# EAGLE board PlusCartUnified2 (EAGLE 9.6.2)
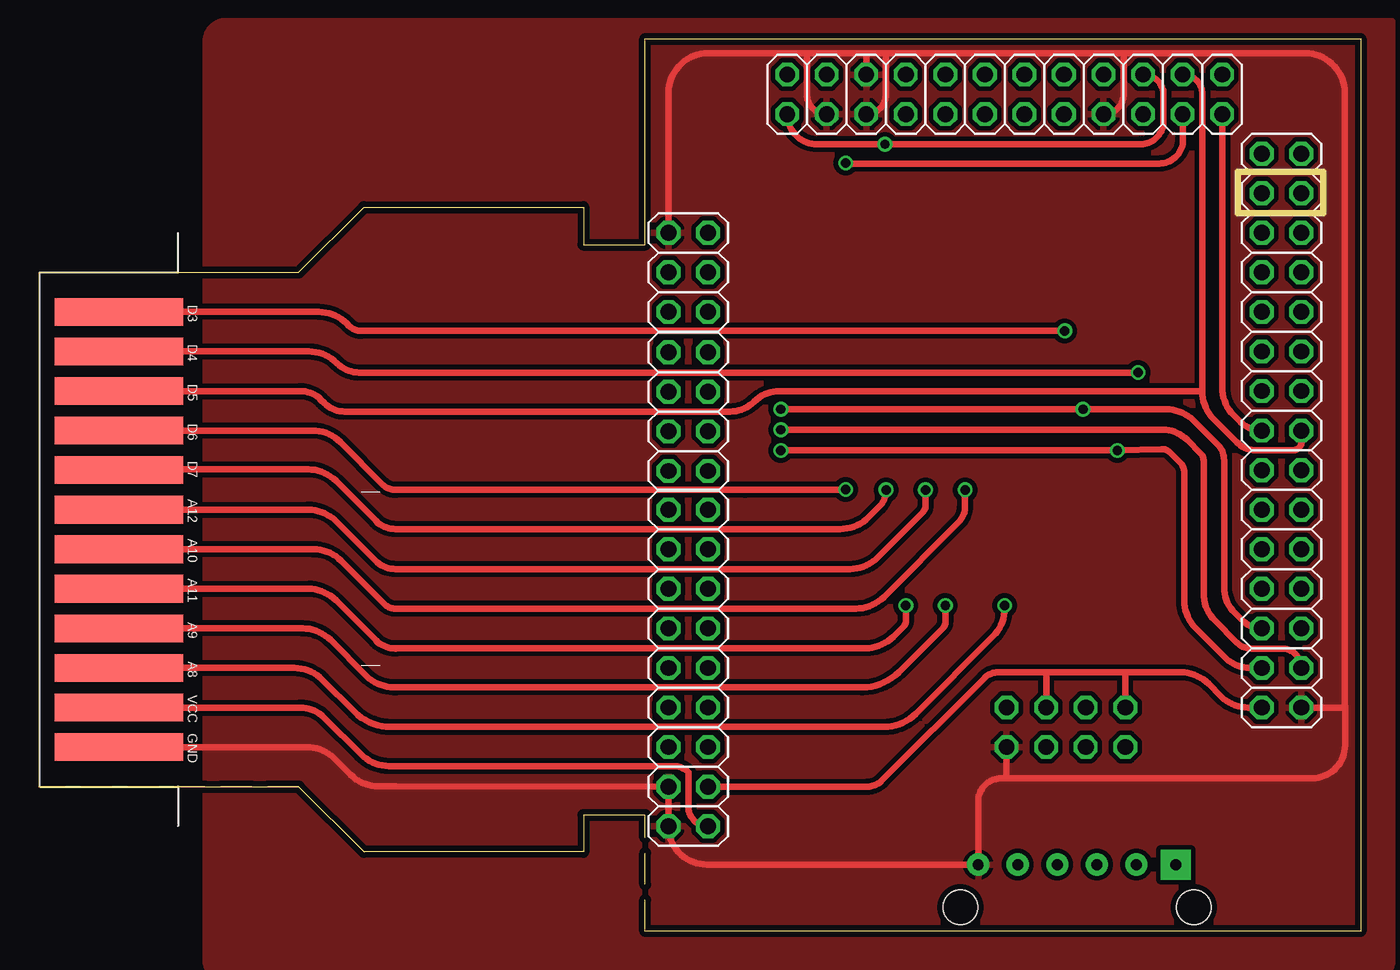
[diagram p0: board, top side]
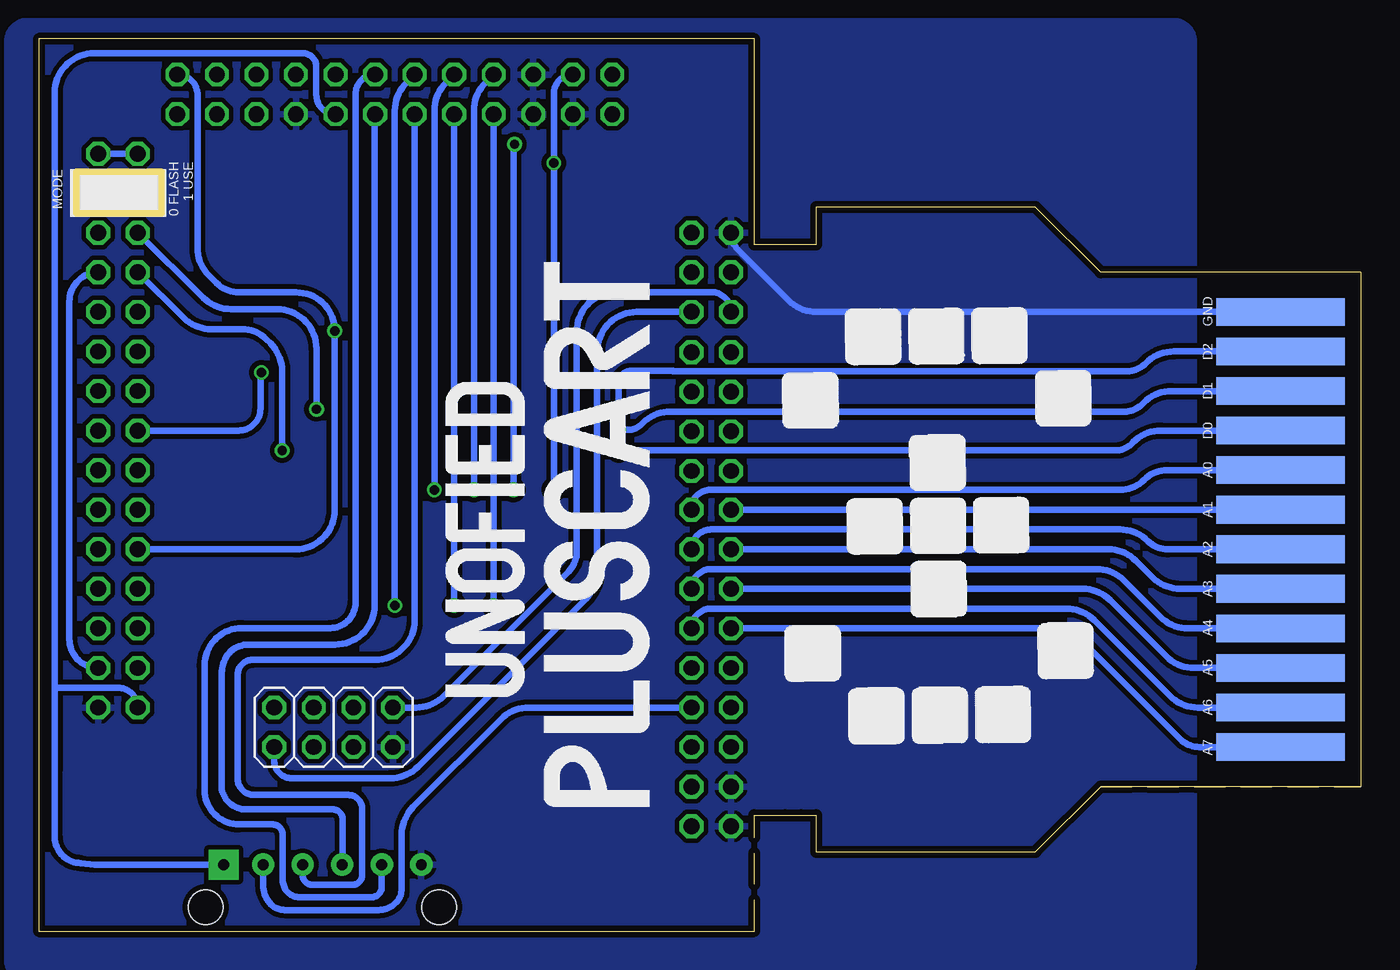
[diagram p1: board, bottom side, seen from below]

Size 84.89 x 57.28 mm. Coordinates in mm from the lower left corner, seen from the top.
Outline: 38.94,7.44 34.98,7.44
Outline: 34.98,7.44 34.98,5.08 20.88,5.08 16.69,9.27
Outline: 0,9.27 0,42.29 16.69,42.29 20.88,46.48 34.98,46.48 34.98,44.07 38.94,44.07 38.94,57.28 84.89,57.28 84.89,0 38.94,0 38.94,7.44
Outline: 0,9.27 16.69,9.27
Outline: 38.94,7.44 34.98,7.44
Outline: 16.69,9.27 0,9.27
Copper layers (1*16): Top 0.0356mm / dielectric 1.5011mm / Bottom 0.0356mm
Design rules "OSHPark2layer": minimum track width 6mil, minimum drill 13mil, track to track 6mil, track to pad 6mil, pad to pad 6mil, via to via 6mil, smd to smd 6mil, copper to edge 15mil, drill to drill 6mil, minimum pad ring 7mil, minimum via ring 7mil, stop-mask expansion 3mil, vias tented up to drill 0mil, thermal gap 10mil
Milling: 4 lines

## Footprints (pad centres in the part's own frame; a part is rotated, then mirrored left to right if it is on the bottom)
24PINEDGE-254MM = smd 1.778 x 8.255: 1-A -22.86,-7.62; 2-A -20.32,-7.62; 3-A -17.78,-7.62; 4-A -15.24,-7.62; 5-A -12.7,-7.62; 6-A -10.16,-7.62; 7-A -7.62,-7.62; 8-A -5.08,-7.62; 9-A -2.54,-7.62; 10-A 0,-7.62; 11-A 2.54,-7.62; 12-A 5.08,-7.62 | smd 1.778 x 8.255 bottom: 1-B -22.86,-7.62; 2-B -20.32,-7.62; 3-B -17.78,-7.62; 4-B -15.24,-7.62; 5-B -12.7,-7.62; 6-B -10.16,-7.62; 7-B -7.62,-7.62; 8-B -5.08,-7.62; 9-B -2.54,-7.62; 10-B 0,-7.62; 11-B 2.54,-7.62; 12-B 5.08,-7.62
2X02 = drill 1.016 octagon: 1 -1.27,-1.27; 2 -1.27,1.27; 3 1.27,-1.27; 4 1.27,1.27
2X04 = drill 1.016 octagon: 1 -3.81,-1.27; 2 -3.81,1.27; 3 -1.27,-1.27; 4 -1.27,1.27; 5 1.27,-1.27; 6 1.27,1.27; 7 3.81,-1.27; 8 3.81,1.27
2X03 = drill 1.016 octagon: 1 -2.54,-1.27; 2 -2.54,1.27; 3 0,-1.27; 4 0,1.27; 5 2.54,-1.27; 6 2.54,1.27
2X09 = drill 1.016 octagon: 1 -10.16,-1.27; 2 -10.16,1.27; 3 -7.62,-1.27; 4 -7.62,1.27; 5 -5.08,-1.27; 6 -5.08,1.27; 7 -2.54,-1.27; 8 -2.54,1.27; 9 0,-1.27; 10 0,1.27; 11 2.54,-1.27; 12 2.54,1.27; 13 5.08,-1.27; 14 5.08,1.27; 15 7.62,-1.27; 16 7.62,1.27; 17 10.16,-1.27; 18 10.16,1.27
2X08 = drill 1.016 octagon: 1 -8.89,-1.27; 2 -8.89,1.27; 3 -6.35,-1.27; 4 -6.35,1.27; 5 -3.81,-1.27; 6 -3.81,1.27; 7 -1.27,-1.27; 8 -1.27,1.27; 9 1.27,-1.27; 10 1.27,1.27; 11 3.81,-1.27; 12 3.81,1.27; 13 6.35,-1.27; 14 6.35,1.27; 15 8.89,-1.27; 16 8.89,1.27
2X07 = drill 1.016 octagon: 1 -7.62,-1.27; 2 -7.62,1.27; 3 -5.08,-1.27; 4 -5.08,1.27; 5 -2.54,-1.27; 6 -2.54,1.27; 7 0,-1.27; 8 0,1.27; 9 2.54,-1.27; 10 2.54,1.27; 11 5.08,-1.27; 12 5.08,1.27; 13 7.62,-1.27; 14 7.62,1.27
MICROSD_FOOTPRINT = drill 0.7 pad 1.93 square: 3V3 -15.24,6.35 | drill 0.7 pad 1.422: CLK -15.24,-1.27; CS -15.24,3.81; GND -15.24,-6.35; MISO -15.24,-3.81; MOSI -15.24,1.27 | hole 2.2: -12.5,7.5; -12.5,-7.5

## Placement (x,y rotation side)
CON3  A2600  [24PINEDGE-254MM]  12.75,34.67 90 bottom
JP1  0  [2X02]  41.71,8 270 top
JP2  0  [2X04]  41.71,23.24 270 top
JP3  0  [2X03]  41.71,42.29 270 top
JP4  0  [2X09]  58.22,53.72 180 top
JP5  0  [2X08]  79.81,23.24 90 top
JP6  0  [2X04]  65.96,13.08 0 bottom
JP7  0  [2X03]  41.71,14.35 270 top
JP8  0  [2X04]  41.71,33.35 270 top
JP10  0  [2X03]  73.46,53.72 0 top
JP11  0  [2X07]  79.81,42.29 270 top
SD1  MICROSDMICROSD2  [MICROSD_FOOTPRINT]  66.68,-10.97 270 top

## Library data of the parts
CON3 = con-edge
JP1-JP6 = pinhead
JP7 JP8 JP10 JP11 = pinhead@1
SD1 = MICROSD

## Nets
+3V3: JP1.2 JP4.4 JP5.2 JP6.2 JP6.6 SD1.3V3
A0: CON3.8-A JP2.2
A1: CON3.7-A JP2.1
A2: CON3.6-A JP2.4
A3: CON3.5-A JP2.3
A4: CON3.4-A JP2.6
A5: CON3.3-A JP2.5
A6: CON3.2-A JP2.8
A7: CON3.1-A JP2.7
A8: CON3.3-B JP4.7
A9: CON3.4-B JP4.10
A10: CON3.6-B JP4.9
A11: CON3.5-B JP4.12
A12: CON3.7-B JP4.11
CLK: JP4.6 SD1.CLK
CS: JP7.4 SD1.CS
D0: CON3.9-A JP5.4 JP11.7
D1: CON3.10-A JP5.3 JP11.8
D2: CON3.11-A JP5.6 JP11.5
D3: CON3.12-B JP5.10 JP10.6
D4: CON3.11-B JP5.16 JP10.5
D5: CON3.10-B JP5.15 JP10.4
D6: CON3.9-B JP4.15 JP10.3
D7: CON3.8-B JP4.18 JP10.2
GND: CON3.1-B CON3.12-A JP1.1 JP1.3 JP3.1 JP4.2 JP4.13 JP4.14 JP4.16 JP5.1 JP6.7 SD1.GND
MISO: JP4.5 SD1.MISO
MOSI: JP4.8 SD1.MOSI
SHORT: JP11.1 JP11.2
USART1_RX: JP3.5 JP6.8
USART1_TX: JP3.6 JP6.1
VCC: CON3.2-B JP1.4

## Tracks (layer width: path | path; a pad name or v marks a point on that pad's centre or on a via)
+3V3
  Top 0.406: JP1.2 53.22,9.27 arc45 54.12,9.64 60.71,16.24 arc-45 61.61,16.61 64.78,16.61 | JP5.2 77.67,14.35 arc-45 75.92,15.07 75.13,15.87 arc45 73.33,16.61 69.84,16.61 | 64.78,16.61 69.84,16.61 | JP6.6 64.69,16.39 arc-45 64.78,16.61 | JP6.2 69.77,16.44 arc-45 69.84,16.61
  Bottom 0.406: JP4.4 arc90 67.07,53.68 67.07,55.5 arc-90 67.94,56.37 81.33,56.37 arc-90 83.87,53.83 83.87,15.62 | 83.87,15.62 83.87,10.37 arc90 83.86,10.36 83.86,6.02 arc-90 82.21,4.37 81.3,4.27 SD1.3V3 | JP5.2 arc-90 79.81,15.62 83.87,15.62
A0
  Bottom 0.406: JP2.2 42.98,27.12 arc90 41.77,28.33 15.47,28.33 arc-45 13.89,28.98 arc45 12.42,29.59 CON3.8-A
A1
  Bottom 0.406: JP2.1 CON3.7-A
A2
  Bottom 0.406: JP2.4 arc90 41.71,25.78 15.45,25.78 arc45 13.66,25.04 arc-45 12.39,24.51 CON3.6-A
A3
  Bottom 0.406: JP2.3 16.22,24.51 arc45 14.42,23.77 13.37,22.71 arc-45 11.57,21.97 CON3.5-A
A4
  Bottom 0.406: JP2.6 arc90 41.71,23.24 16.98,23.24 arc45 15.18,22.5 12.86,20.18 arc-45 11.06,19.43 CON3.4-A
A5
  Bottom 0.406: JP2.5 17.87,21.97 arc45 16.07,21.23 12.48,17.64 arc-45 10.68,16.89 CON3.3-A
A6
  Bottom 0.406: JP2.8 arc90 41.71,20.7 18.91,20.7 arc45 17.11,19.96 12.25,15.1 arc-45 10.45,14.35 CON3.2-A
A7
  Bottom 0.406: JP2.7 19.75,19.43 arc45 17.95,18.69 11.58,12.32 arc-45 10.36,11.81 CON3.1-A
A8  (via drill 0.6)
  Top 0.406: CON3.3-B 16.4,16.89 arc-45 18.19,16.15 20.26,14.08 arc45 22.6,13.11 54.28,13.11 arc45 56.32,13.95 61.28,18.92 arc45 62.03,20.71 v62.03,20.9
  Bottom 0.406: JP4.7 61.28,54.47 arc-45 62.03,52.67 v62.03,20.9
A9  (via drill 0.6)
  Top 0.406: v58.22,20.9 58.22,19.84 arc-45 58.05,19.45 55.23,16.62 arc-45 52.89,15.65 22.91,15.65 22.82,15.65 arc-45 21.02,16.39 18.73,18.69 arc45 16.93,19.43 CON3.4-B
  Bottom 0.406: JP4.10 v58.22,20.9
A10  (via drill 0.6)
  Top 0.406: v59.49,28.32 59.49,27.28 arc-45 59.06,26.24 54.26,21.45 arc-45 52.47,20.7 22.91,20.7 arc-45 22.17,21.01 19.41,23.77 arc45 17.62,24.51 CON3.6-B
  Bottom 0.406: JP4.9 58.74,54.47 arc-45 59.49,52.67 v59.49,28.32
A11  (via drill 0.6)
  Top 0.406: v55.68,20.9 55.68,19.89 arc-45 55.55,19.59 54.87,18.91 arc-45 53.07,18.16 22.97,18.16 arc45 22.91,18.14 arc-45 21.65,18.66 19.08,21.23 arc45 17.29,21.97 CON3.5-B
  Bottom 0.406: JP4.12 v55.68,20.9
A12  (via drill 0.6)
  Top 0.406: v56.95,28.32 56.95,27.33 arc-45 56.75,26.85 53.88,23.98 arc-45 52.08,23.24 22.91,23.24 arc-45 21.61,23.78 19.08,26.31 arc45 17.29,27.05 CON3.7-B
  Bottom 0.406: JP4.11 56.2,54.47 arc-45 56.95,52.67 v56.95,28.32
CLK
  Bottom 0.406: JP4.6 arc-45 63.32,52.4 63.32,20.93 arc90 65.86,18.39 71.42,18.39 arc-90 73.11,16.71 arc-90 73.16,16.65 73.16,9.39 arc-90 71.59,7.81 66.01,7.81 arc90 65.38,7.18 65.38,4.29 arc90 SD1.CLK
CS
  Bottom 0.406: JP7.4 53.41,14.35 arc-45 55.21,13.61 60.85,7.97 arc-45 61.59,6.17 61.59,2.72 arc45 61.97,1.81 arc45 63.08,1.35 69.11,1.35 arc45 69.97,1.7 arc45 70.48,2.95 SD1.CS
D0  (via drill 0.6)
  Top 0.406: JP5.4 77.76,16.89 arc-45 76.23,17.53 74.3,19.45 arc-45 73.56,21.25 73.56,29.47 arc45 73.31,30.07 72.64,30.73 arc45 72.13,30.95 v69.27,30.85 v47.65,30.85
  Bottom 0.406: v47.65,30.85 15.77,30.85 arc-45 14.71,31.29 14.61,31.39 arc45 12.82,32.13 CON3.9-A | JP11.7 75.58,39.38 arc-45 73.79,38.63 71.81,38.63 arc45 70.28,38 70.01,37.73 arc45 69.27,35.93 v69.27,30.85
D1  (via drill 0.6)
  Top 0.406: JP5.3 arc90 79.83,18.14 77.9,18.14 arc-45 76.9,18.55 75.55,19.91 arc-45 74.8,21.7 74.8,30.23 arc45 74.62,30.66 73.75,31.54 arc45 72.19,32.18 v47.65,32.18
  Bottom 0.406: JP5.3 arc90 82.93,18.74 82.93,40.41 arc90 JP11.8 | CON3.10-A 12.13,34.67 arc-45 13.93,33.93 14.02,33.83 arc45 15.19,33.35 44.31,33.35 arc-45 46.11,32.61 46.18,32.54 arc45 47.04,32.18 v47.65,32.18
D2  (via drill 0.6)
  Top 0.406: v47.65,33.5 v67.06,33.5 72.38,33.5 arc-45 74.18,32.76 75.72,31.22 arc-45 76.12,30.23 76.12,22.08 arc45 76.81,20.42 77.28,19.95 arc45 JP5.6
  Bottom 0.406: JP11.5 74.34,40.67 arc-45 72.54,39.93 69.6,39.93 arc90 67.06,37.39 v67.06,33.5 | v47.65,33.5 47.65,35.18 arc90 46.86,35.97 44.18,35.97 arc90 44.16,35.94 14.97,35.94 arc-45 13.87,36.4 13.8,36.47 arc45 12,37.21 CON3.11-A
D3  (via drill 0.6)
  Top 0.406: v65.89,38.53 20.67,38.53 arc-45 19.94,38.84 19.77,39.01 arc45 17.97,39.75 CON3.12-B
  Bottom 0.406: JP5.10 68.42,24.51 arc-90 65.88,27.05 65.88,38.51 arc-45 v65.89,38.53 arc-90 68.36,41.01 72.03,41.01 arc45 73.49,41.61 73.96,42.08 arc45 74.7,43.88 74.7,53.66 arc-90 JP10.6
D4  (via drill 0.6)
  Top 0.406: JP5.16 arc-45 77.15,32.71 76.74,33.11 arc-45 76,34.91 76,35.93 arc45 76.02,35.98 JP10.5 | v70.6,35.86 20.58,35.86 arc-45 19.15,36.45 19.13,36.47 arc45 17.34,37.21 CON3.11-B
  Bottom 0.406: JP5.16 72.07,32.13 arc-90 70.66,33.54 70.66,35.8 arc90 v70.6,35.86
D5
  Top 0.406: JP10.4 arc-90 74.73,53.74 74.73,34.69 arc-90 74.71,34.67 | 74.71,34.67 74.71,34.66 arc45 75.46,32.87 76.95,31.38 arc45 78.16,30.88 80.55,30.88 arc90 81.1,31.43 81.1,32.11 arc90 JP5.15 | 74.71,34.67 47.58,34.67 arc45 45.92,33.99 arc-45 44.39,33.35 19.63,33.35 arc-45 18.34,33.88 18.11,34.11 arc45 16.76,34.67 CON3.10-B
D6  (via drill 0.6)
  Top 0.406: v51.82,28.35 45.39,28.35 45.36,28.32 22.91,28.32 arc-45 22.09,28.66 19.36,31.39 arc45 17.57,32.13 CON3.9-B | JP10.3 73.48,50.81 arc-90 71.95,49.28 51.86,49.28 arc-90 v51.82,49.32
  Bottom 0.406: v51.82,28.35 v51.82,49.32 51.82,53.77 arc90 JP4.15
D7  (via drill 0.6)
  Top 0.406: v54.41,28.32 arc-45 53.96,27.24 53.29,26.57 arc-45 51.45,25.81 22.91,25.81 arc-45 21.65,26.33 19.08,28.9 arc45 17.29,29.64 5.25,29.64 arc45 CON3.8-B | JP4.18 arc90 49.99,50.52 v54.34,50.52 70.76,50.52 arc90 72.23,51.99 72.23,53.7 arc90 JP10.2
  Bottom 0.406: v54.41,28.32 54.41,50.45 arc-90 v54.34,50.52
GND
  Top 0.406: 83.87,14.45 83.87,53.82 arc90 81.33,56.36 69.68,56.36 | 69.68,56.36 54.41,56.36 | 54.41,56.36 53.19,56.36 | JP4.2 arc90 69.68,53.75 69.68,56.36 | JP3.1 40.44,53.82 arc-90 42.98,56.36 49.33,56.36 | 49.33,56.36 53.19,56.36 | JP4.13 53.14,56.3 arc-90 53.19,56.36 | JP4.16 arc-90 49.33,53.72 49.33,56.36 | JP4.14 arc90 54.41,53.72 54.41,56.36 | CON3.1-B 17.18,11.81 arc-45 18.98,11.07 20.01,10.04 arc45 21.8,9.3 22.91,9.3 JP1.1 JP1.3 arc90 42.9,4.27 SD1.GND 60.32,8.31 arc-90 61.83,9.81 62.18,9.81 | JP6.7 62.15,9.84 arc90 62.18,9.81 | 83.87,14.45 arc-90 83.89,14.42 83.89,11.93 arc-90 81.77,9.81 62.18,9.81 | JP5.1 83.77,14.35 arc90 83.87,14.45
  Bottom 0.406: JP3.1 arc-45 39.99,43.75 36.74,40.5 arc-45 34.94,39.75 CON3.12-A
  pour Top (isolate 0.305): 10.72,-1.91 10.72,57.15 arc-90 11.99,58.42 86.92,58.42 86.92,-1.91 arc-90 85.65,-3.17 11.99,-3.17 arc-90
  pour Bottom (isolate 0.305): 10.72,57.15 10.72,-1.91 arc90 11.99,-3.17 85.65,-3.17 arc90 86.92,-1.91 86.92,57.15 arc90 85.65,58.42 11.99,58.42 arc90
MISO
  Bottom 0.406: JP4.5 arc-90 64.55,53.74 64.55,21.09 arc90 66.19,19.45 71.84,19.45 arc-90 74.24,17.05 74.24,9 arc-45 73.63,7.54 73.59,7.49 arc-45 72.04,6.85 69.89,6.85 arc90 69.22,6.18 69.22,3.25 arc-90 68.14,2.17 63.53,2.17 arc-90 62.86,2.85 SD1.MISO arc-90 SD1.MISO
MOSI
  Bottom 0.406: JP4.8 60.76,19.95 arc90 63.3,17.41 71.17,17.41 arc-90 72.12,16.46 72.12,9.79 arc-90 71.07,8.74 65.03,8.74 arc90 64.12,7.83 64.12,5.73 | 64.12,5.73 64.12,3.59 arc90 64.73,2.98 67.34,2.98 arc90 67.94,3.58 SD1.MOSI | 64.12,5.73
SHORT
  Bottom 0.406: JP11.1 JP11.2
USART1_RX
  Bottom 0.406: JP3.5 arc-90 41.71,41.02 47.8,41.02 arc-90 50.34,38.48 50.34,24.38 arc45 50.88,23.08 58.87,15.1 arc45 60.67,14.35 JP6.8
USART1_TX
  Bottom 0.406: JP3.6 46.49,39.75 arc-90 49.03,37.21 49.03,24.23 arc45 49.05,24.19 49.05,23.09 arc45 49.79,21.29 60.53,10.56 arc45 62.32,9.81 68.65,9.81 arc90 69.77,10.94 JP6.1
VCC
  Top 0.406: JP1.4 arc-90 41.71,8 arc45 41.71,8 41.71,10.2 arc45 40.77,10.59 22.91,10.59 22.49,10.59 arc-45 20.69,11.34 18.32,13.7 arc45 16.76,14.35 CON3.2-B

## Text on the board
tNames: D3 | D4 | D5 | D6 | D7 | A12 | A10 | A11 | A9 | A8 | VCC | GND
bNames: 0 FLASH / 1 USE | MODE | GND | D2 | D1 | D0 | A0 | A1 | A2 | A3 | A4 | A5 | A6 | A7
